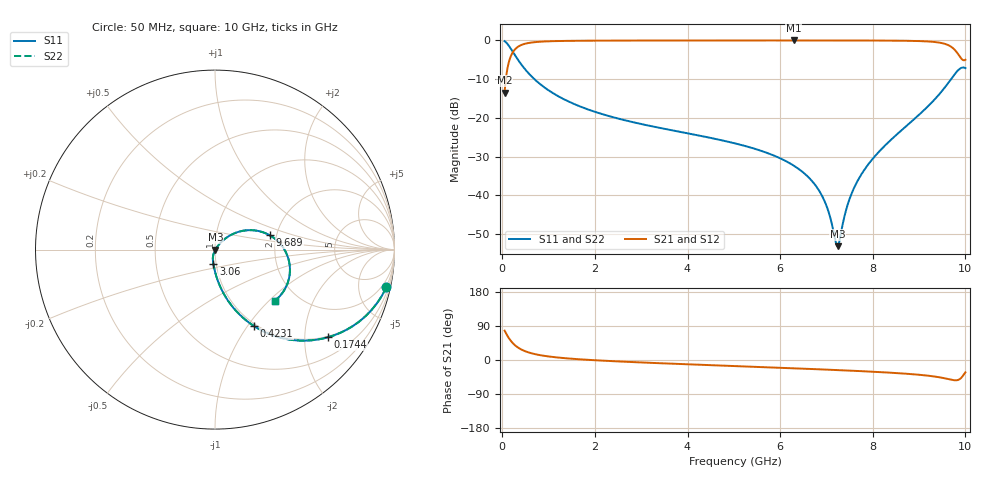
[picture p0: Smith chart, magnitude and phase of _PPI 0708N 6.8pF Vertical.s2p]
! S-Parameter data specifications (vertical orientation):
! Substrate: 40-mil Rogers 3003C, Substrate thickness, H=1.016mm, Dielectric constant, Er=3, Conductor thickness, T_mtl=0.043mm, Loss Tangent, Tand=0.003
! PCB Mounting Pad Footprint: Pad width, PadW=2.54mm , Pad length, PadL=0.51mm , Pad gap, PadG (edge-to-edge)=0.71mm , Reference planes=1.73mm apart
! Created Tue Jan 16 08:46:16 2018
# GHz S MA R 50
! 2 Port Network Data from SP1.SP block
! freq  magS11  angS11  magS21  angS21  magS12  angS12  magS22  angS22
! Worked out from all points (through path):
!   801 points, 50 MHz to 10 GHz, reference 50 ohm
!   highest |S21| = -0.02 dB at 6.294 GHz (marker M1); lowest = -13.4 dB at 50 MHz (marker M2)
!   group delay of S21, straight-line fit = 18.6 ps
!   lowest |S11| = -53.1 dB at 7.239 GHz (marker M3), VSWR 1.00, Z = 50.2 - j0.103 ohm
!   |S11| at or under -10 dB: 693.6 MHz to 9.689 GHz (8.996 GHz wide, 173 % of centre)
!   |S22| runs from -53.1 to -0.2 dB; largest |S21 - S12| = 0
!   S11 on the Smith chart (normalised r, x): 50 MHz: 0.97, -9.05; 174.4 MHz: 0.97, -2.60; 423.1 MHz: 0.97, -1.07; 3.06 GHz: 0.97, -0.16; 9.689 GHz: 1.84, +0.33; 10 GHz: 1.54, -1.09
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0.05  0.9771 -12.5  0.2127 77.5  0.2127 77.5  0.9771 -12.5
0.174375  0.7964 -37.8  0.6045 52.1  0.6045 52.1  0.7964 -37.8
0.2863125  0.626 -52.3  0.7795 37.7  0.7795 37.7  0.626 -52.3
0.423125  0.4779 -63.0  0.8781 26.9  0.8781 26.9  0.4779 -63.0
0.821125  0.2717 -77.2  0.9619 12.7  0.9619 12.7  0.2717 -77.2
1.716625  0.1378 -88.3  0.9898 1.5  0.9898 1.5  0.1378 -88.3
3.059875  0.08195 -96.2  0.9957 -6.8  0.9957 -6.8  0.08195 -96.2
3.370812  0.07499 -97.7  0.9962 -8.3  0.9962 -8.3  0.07499 -97.7
5.025  0.04697 -104.6  0.9976 -16.0  0.9976 -16.0  0.04697 -104.6
6.293625  0.02425 -108.3  0.9979 -21.9  0.9979 -21.9  0.02425 -108.3
6.691625  0.01525 -107.2  0.9979 -23.8  0.9979 -23.8  0.01525 -107.2
6.977688  0.007957 -101.0  0.9977 -25.2  0.9977 -25.2  0.007957 -101.0
7.238875  0.002218 -27.7  0.9975 -26.6  0.9975 -26.6  0.002218 -27.7
7.288625  0.002743 7.1  0.9974 -26.9  0.9974 -26.9  0.002743 7.1
7.46275  0.007781 43.4  0.9972 -27.8  0.9972 -27.8  0.007781 43.4
7.636875  0.01406 49.8  0.9968 -28.8  0.9968 -28.8  0.01406 49.8
7.922937  0.0261 52.0  0.9959 -30.5  0.9959 -30.5  0.0261 52.0
8.345812  0.04911 50.8  0.9934 -33.2  0.9934 -33.2  0.04911 50.8
9.228875  0.1484 39.1  0.9656 -41.9  0.9656 -41.9  0.1484 39.1
9.689063  0.3161 14.5  0.8301 -51.8  0.8301 -51.8  0.3161 14.5
9.863188  0.4234 -11.1  0.6388 -51.5  0.6388 -51.5  0.4234 -11.1
10  0.4388 -40.5  0.5632 -32.6  0.5632 -32.6  0.4388 -40.5
